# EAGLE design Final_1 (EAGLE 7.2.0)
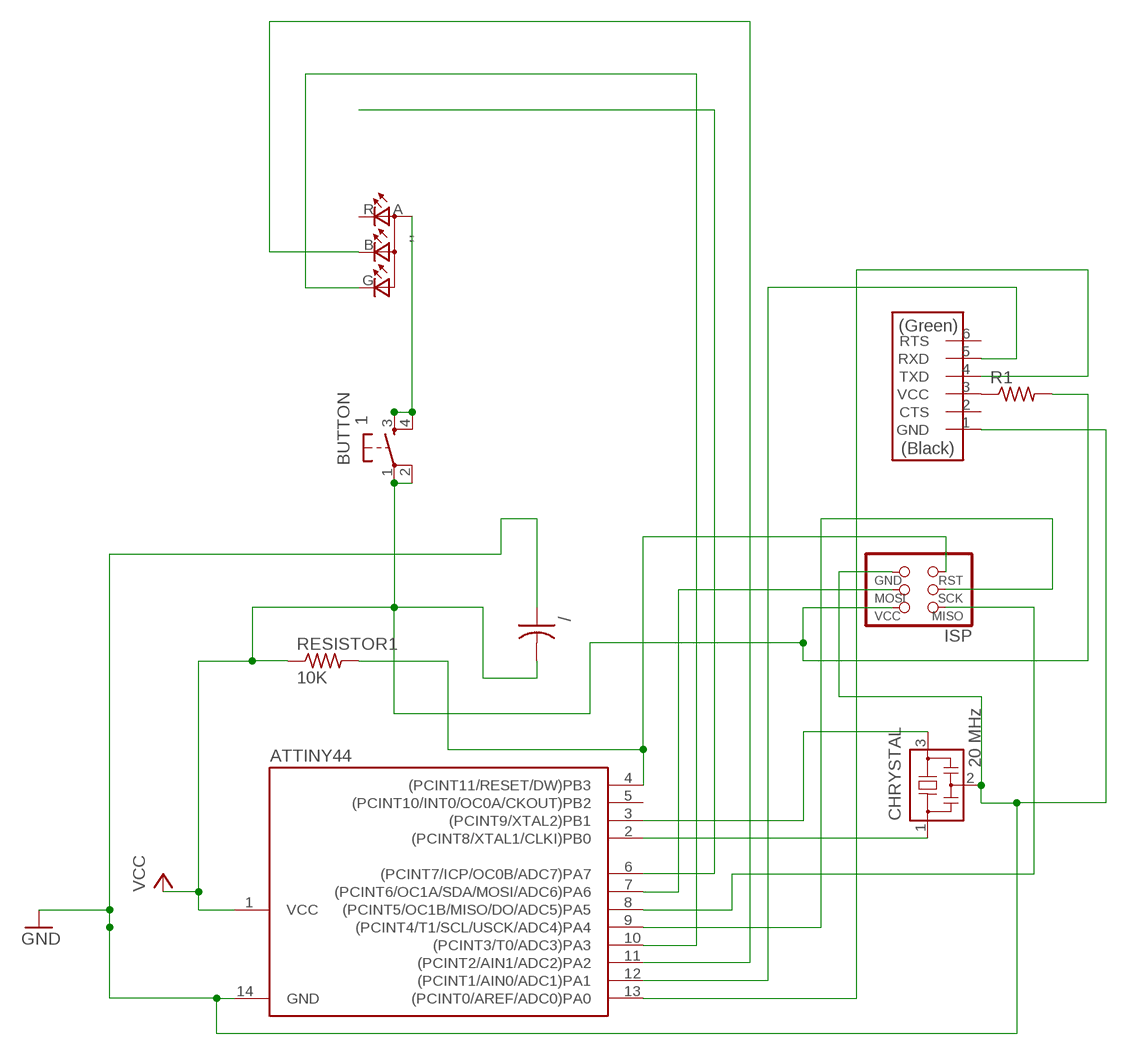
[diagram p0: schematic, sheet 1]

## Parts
,,  LEDRGBNEW  [P-LCC-4]
/  CAP-US1206FAB  [C1206FAB]
ATTINY44  ATTINY44-SSU  [SOIC14]
BUTTON  1  6MM_SWITCH6MM_SWITCH  [6MM_SWITCH]
CHRYSTAL  20 MHz  RESONATOR  [EFOBM]
ISP  AVRISPSMD  [2X03SMD]
PIN  FTDI-SMD-HEADER  [1X06SMD]
R1  RES-US1206FAB  [R1206FAB]
RESISTOR1  10K  RES-US1206FAB  [R1206FAB]

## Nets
GND: /.1 ATTINY44.14(GND) CHRYSTAL.2 ISP.6(GND) PIN.1(GND)
N$1: PIN.3(VCC) R1.1
N$2: ATTINY44.2((PCINT8/XTAL1/CLKI)PB0) CHRYSTAL.1
N$3: ATTINY44.3((PCINT9/XTAL2)PB1) CHRYSTAL.3
N$4: ATTINY44.6((PCINT7/ICP/OC0B/ADC7)PA7)
N$5: ATTINY44.13((PCINT0/AREF/ADC0)PA0) PIN.4(TXD)
N$6: ATTINY44.12((PCINT1/AIN0/ADC1)PA1) PIN.5(RXD)
N$7: ATTINY44.4((PCINT11/RESET/DW)PB3) ISP.5(RST) RESISTOR1.2
N$8: ATTINY44.9((PCINT4/T1/SCL/USCK/ADC4)PA4) ISP.3(SCK)
N$9: ATTINY44.7((PCINT6/OC1A/SDA/MOSI/ADC6)PA6) ISP.4(MOSI)
N$10: ATTINY44.8((PCINT5/OC1B/MISO/DO/ADC5)PA5) ISP.1(MISO)
N$11: ,,.A(A2) BUTTON.3(S) BUTTON.4(S1)
N$13: ,,.B(CBLUE) ATTINY44.11((PCINT2/AIN1/ADC2)PA2)
N$14: ,,.G(CGREEN) ATTINY44.10((PCINT3/T0/ADC3)PA3)
VCC: /.2 ATTINY44.1(VCC) BUTTON.1(P) BUTTON.2(P1) ISP.2(VCC) R1.2 RESISTOR1.1
Unconnected: ,,.R(CRED) ATTINY44.5((PCINT10/INT0/OC0A/CKOUT)PB2) PIN.2(CTS) PIN.6(RTS)

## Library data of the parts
,, = fab:LEDRGBNEW
/ = fab:CAP-US
ATTINY44 = fab:ATTINY44
BUTTON = fab:6MM_SWITCH: OMRON SWITCH
CHRYSTAL = fab:RESONATOR
ISP = fab:AVRISP
PIN = fab:FTDI-SMD-HEADER
R1 RESISTOR1 = fab:RES-US: Resistor (US Symbol)

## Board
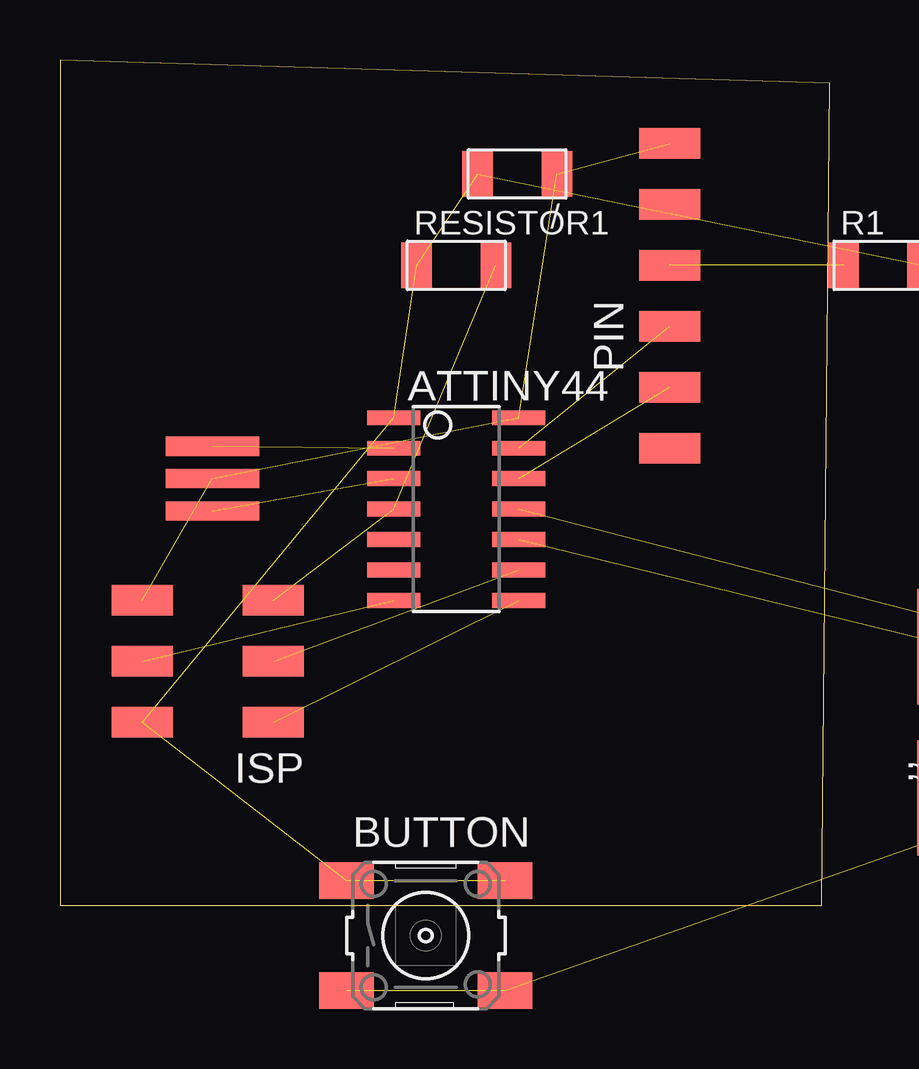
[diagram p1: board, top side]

Size 32.08 x 35.23 mm. Coordinates in mm from the lower left corner, seen from the top.
Outline: 0,0 31.73,0 32.08,34.27 0,35.23 0,0
Copper layers (1*16): Top 0.035mm / dielectric 1.5mm / Bottom 0.035mm
Design rules "default": minimum track width 10mil, minimum drill 24mil, track to track 8mil, track to pad 8mil, pad to pad 8mil, via to via 8mil, smd to smd 8mil, copper to edge 40mil, drill to drill 8mil, minimum pad ring 10mil, minimum via ring 8mil, stop-mask expansion 4mil, vias tented up to drill 0mil, thermal gap 10mil

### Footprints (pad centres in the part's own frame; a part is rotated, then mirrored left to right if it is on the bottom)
P-LCC-4 = smd 3.3 x 4.8: A 2,-3.15; B 2,3.15; G -2,3.15; R -2,-3.15
C1206FAB = smd 1.27 x 1.905: 1 -1.651,0; 2 1.651,0
SOIC14 = smd 0.61 x 2.21: 1 -3.81,-2.603; 2 -2.54,-2.603; 3 -1.27,-2.603; 4 0,-2.603; 5 1.27,-2.603; 6 2.54,-2.603; 7 3.81,-2.603; 8 3.81,2.603; 9 2.54,2.603; 10 1.27,2.603; 11 0,2.603; 12 -1.27,2.603; 13 -2.54,2.603; 14 -3.81,2.603
6MM_SWITCH = smd 2.286 x 1.524: 1 -3.302,2.286; 2 3.302,2.286; 3 -3.302,-2.286; 4 3.302,-2.286
EFOBM = smd 0.8 x 3.9: 1 -1.35,0; 2 0,0; 3 1.35,0
2X03SMD = smd 2.54 x 1.27: 1 -2.54,2.54; 2 2.92,2.54; 3 -2.54,0; 4 2.92,0; 5 -2.54,-2.54; 6 2.92,-2.54
1X06SMD = smd 2.54 x 1.27: 1 0,6.35; 2 0,3.81; 3 0,1.27; 4 0,-1.27; 5 0,-3.81; 6 0,-6.35
R1206FAB = smd 1.27 x 1.905: 1 -1.651,0; 2 1.651,0

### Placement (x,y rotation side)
,,  not placed on the board
/  19.05,30.48 180 top
ATTINY44  16.51,16.51 270 top
BUTTON  15.24,-1.27 0 top
CHRYSTAL  6.35,17.78 270 top
ISP  6.35,10.16 180 top
PIN  25.4,25.4 0 top
R1  34.29,26.67 0 top
RESISTOR1  16.51,26.67 0 top

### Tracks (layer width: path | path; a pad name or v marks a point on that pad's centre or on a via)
GND  (4 unrouted)
N$1  (1 unrouted)
N$2  (1 unrouted)
  Top 0.406: 13.91,19.13 ATTINY44.2
N$3  (1 unrouted)
N$5  (1 unrouted)
N$6  (1 unrouted)
N$7  (2 unrouted)
N$8  (1 unrouted)
N$9  (1 unrouted)
N$10  (1 unrouted)
N$11  (2 unrouted)
N$13  (1 unrouted)
N$14  (1 unrouted)
VCC  (6 unrouted)

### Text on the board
Top: When FAB12?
